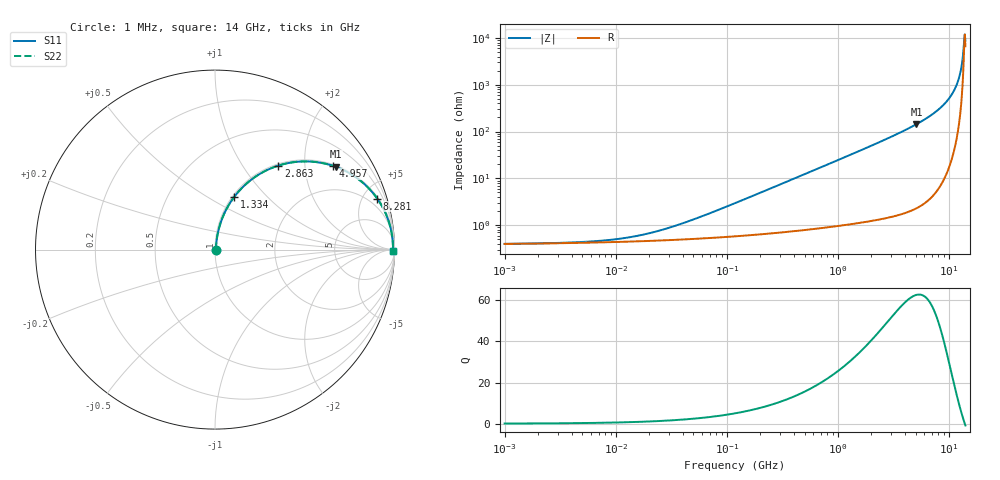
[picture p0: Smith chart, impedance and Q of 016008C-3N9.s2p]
# MHz S MA R 50
!Freq  MagS11  AngS11  MagS21  AngS21  MagS12  AngS12  MagS22  AngS22
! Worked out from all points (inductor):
!   801 points, 1 MHz to 14 GHz, reference 50 ohm
!   read as one part in series: L = 3.9 nH near 65.15 MHz
!   highest Q = 62.7 at 5.077 GHz (marker M1), where L = 4.51 nH
!   self-resonance near 13.67 GHz
!   S11 on the Smith chart (normalised r, x): 1 MHz: 1.01, +0.00; 1.334 GHz: 1.02, +0.66; 2.863 GHz: 1.03, +1.47; 4.957 GHz: 1.04, +2.79; 8.281 GHz: 1.14, +6.33; 14 GHz: open
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1  0.003974 3.5  0.996 -0.0  0.996 -0.0  0.003974 3.5
4.948533  0.004358 16.0  0.9958 -0.1  0.9958 -0.1  0.004358 16.0
11.68498  0.005245 32.8  0.9956 -0.2  0.9956 -0.2  0.005245 32.8
24.19749  0.007528 51.3  0.9953 -0.3  0.9953 -0.3  0.007528 51.3
47.20622  0.01256 65.8  0.9949 -0.7  0.9949 -0.7  0.01256 65.8
119.742  0.02973 77.2  0.9938 -1.7  0.9938 -1.7  0.02973 77.2
585.5183  0.1414 78.6  0.9819 -8.1  0.9819 -8.1  0.1414 78.6
1333.964  0.3105 70.1  0.9407 -18.1  0.9407 -18.1  0.3105 70.1
1977.752  0.4393 62.5  0.8875 -26.0  0.8875 -26.0  0.4393 62.5
2863.085  0.5857 53.0  0.7989 -35.8  0.7989 -35.8  0.5857 53.0
3812.572  0.705 44.2  0.6971 -44.8  0.6971 -44.8  0.705 44.2
4957.202  0.8065 35.3  0.5785 -53.7  0.5785 -53.7  0.8065 35.3
5076.939  0.815 34.5  0.5667 -54.6  0.5667 -54.6  0.815 34.5
6601.163  0.8967 25.3  0.4279 -63.7  0.4279 -63.7  0.8967 25.3
8281.157  0.9477 17.4  0.2994 -71.4  0.2994 -71.4  0.9477 17.4
10143.7  0.977 10.4  0.1815 -77.5  0.1815 -77.5  0.977 10.4
11027.44  0.9844 7.6  0.1326 -79.5  0.1326 -79.5  0.9844 7.6
11705.45  0.9882 5.6  0.09773 -80.3  0.09773 -80.3  0.9882 5.6
12574.31  0.991 3.2  0.05601 -79.1  0.05601 -79.1  0.991 3.2
12878.03  0.9914 2.4  0.04223 -77.1  0.04223 -77.1  0.9914 2.4
13347.42  0.9918 1.2  0.02205 -67.6  0.02205 -67.6  0.9918 1.2
14000  0.9915 -0.4  0.01123 40.7  0.01123 40.7  0.9915 -0.4
